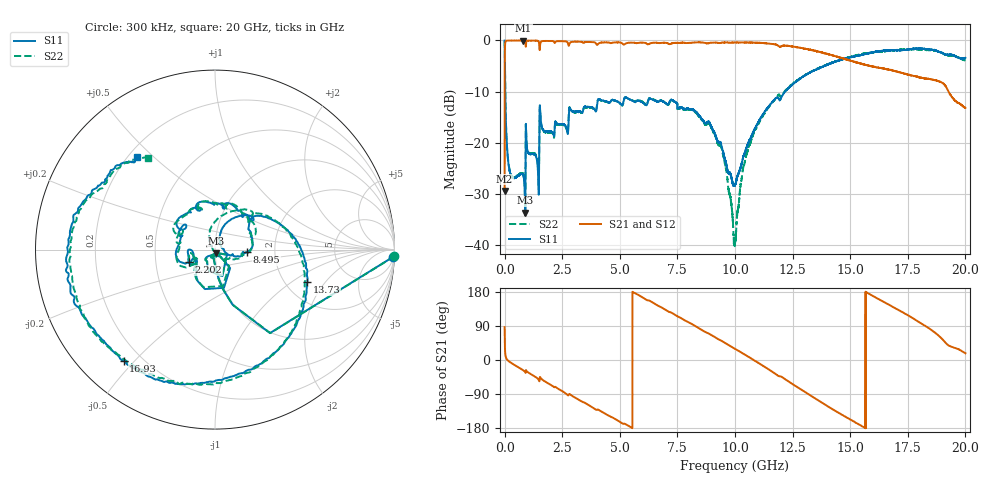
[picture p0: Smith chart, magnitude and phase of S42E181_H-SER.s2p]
! Created Wed Nov 25 22:03:15 2020
# khz S ma R 50
! 2 Port Network Data from SP1.SP block
! freq  magS11  angS11  magS21  angS21  magS12  angS12  magS22  angS22
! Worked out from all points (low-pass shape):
!   20001 points, 300 kHz to 20 GHz, reference 50 ohm
!   highest |S21| = -0.01 dB at 813.3 MHz (marker M1); lowest = -29.5 dB at 300 kHz (marker M2)
!   |S21| within 3 dB of the highest: 8.971 MHz to 14.3 GHz (14.3 GHz wide, 200 % of centre); 14.30714 GHz to 14.30841 GHz (1.261 MHz wide, 0.00882 % of centre)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
!   lowest |S11| = -33.7 dB at 895.3 MHz (marker M3), VSWR 1.04, Z = 50.5 - j2.01 ohm
!   |S11| at or under -10 dB: 26.84 MHz to 12.17 GHz (12.15 GHz wide, 199 % of centre)
!   |S22| runs from -40.2 to 0.0 dB; largest |S21 - S12| = 0.017
!   S11 on the Smith chart (normalised r, x): 300 kHz: 6, -50; 2.202 GHz: 0.74, -0.10; 8.495 GHz: 1.43, -0.04; 13.73 GHz: 2.61, -1.34; 16.93 GHz: 0.13, -0.47; 20 GHz: 0.23, +0.45
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300  0.9951 -2.3  0.03365 86.7  0.03374 87.5  0.9994 -2.2
108300  0.08798 -89.6  0.995 1.1  0.9948 1.1  0.08845 -89.6
285300  0.04761 -101.3  0.9955 -7.7  0.9958 -7.8  0.04834 -101.8
813300  0.04772 -117.6  0.9984 -27.1  0.9969 -27.1  0.0485 -118.6
895300  0.0207 -74.0  0.9838 -32.0  0.9839 -32.0  0.01962 -80.2
2202300  0.1617 -155.2  0.9646 -70.9  0.9646 -70.9  0.1586 -154.4
3334300  0.1998 156.3  0.9675 -109.3  0.968 -109.3  0.1969 167.8
4976300  0.2464 109.9  0.9554 -162.2  0.9546 -162.3  0.2454 109.1
6667300  0.2506 59.3  0.9458 143.0  0.9436 142.9  0.2536 53.9
8495300  0.1771 -4.7  0.9566 81.6  0.9545 81.6  0.1742 -7.4
9437300  0.0893 -20.5  0.9534 49.9  0.9544 49.8  0.08454 -39.0
1.00003e7  0.03888 34.6  0.9546 29.5  0.9564 29.6  0.01084 -155.6
1.03913e7  0.07618 69.7  0.9534 15.4  0.953 15.4  0.06074 121.7
1.09033e7  0.1428 69.0  0.9481 -3.5  0.947 -3.4  0.1362 95.9
1.23083e7  0.3404 31.8  0.8853 -56.2  0.8871 -56.0  0.3467 32.9
1.33343e7  0.4951 -4.3  0.8034 -95.8  0.8078 -95.6  0.4998 -9.5
1.37303e7  0.5438 -19.4  0.7648 -111.1  0.7728 -110.8  0.5494 -24.9
1.54153e7  0.7139 -83.1  0.5955 -171.2  0.5985 -171.9  0.7298 -82.5
1.66673e7  0.7964 -120.9  0.5203 146.6  0.5078 146.8  0.7916 -126.7
1.69263e7  0.8019 -129.4  0.5024 137.8  0.4894 138.2  0.8004 -135.5
1.82643e7  0.8223 -178.2  0.4248 89.8  0.4274 90.5  0.8079 -179.8
2e7  0.6766 129.9  0.218 17.8  0.2189 18.7  0.6314 125.9
